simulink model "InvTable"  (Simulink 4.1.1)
settings: Solver=FixedStepDiscrete  StartTime=0.0  StopTime=inf  FixedStep=samplePeriod  RelTol=1e-3
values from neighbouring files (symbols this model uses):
  aHome = zeros(1, nAct)    [TableInit.m]    (also in displA2T.m = positT2A([0, 0, 0, 0, 0, 0], h); displT2A.m = positT2A([0, 0, 0, 0, 0, 0], h))
  bal = [[ 1 -1 -1  1  0  0  0  0]    [TableInit.m]
  flowCanon = 63090.2    [TableInit.m]    (also in initialize.m)
  gasConstant = 1.8    [TableInit.m]    (also in initialize.m)
  gee = 0    [TableInit.m]    (also in initialize.m = geeCanon / linAccelCanon * ~isempty(find(dof==3)))
  iactParamsX = [actParamsX, dfGain, solver]    [TableInit.m]
  iactParamsY = [actParamsY, dfGain, solver]    [TableInit.m]
  iactParamsZ = [actParamsZ, dfGain, solver]    [TableInit.m]
  inertia = [Ixx 0 0; 0 Iyy 0; 0 0 Izz]    [TableInit.m]    (also in initialize.m = inertia + inertiaP2Q([0 0 0], massA(i), cgA(:,i)-cg,  						)
  inertiaCanon = 0.1130    (= 0.113)    [TableInit.m]    (also in initialize.m = 0.00029264264)
  linAccelCanon = 9.8    [TableInit.m]    (also in accelA2T.m = h(11); accelT2A.m = h(11); Test.m = 9800; initialize.m = 9810)
  linVelocCanon = 10.0    (= 10)    [TableInit.m]    (also in Test.m; initialize.m = 1000)
  mass = 17300    [TableInit.m]    (also in initialize.m = ones(3, 1) * (sum(massA) + massT + massS))
  massCanon = 0.4535924e-06    (= 4.535924e-07)    [TableInit.m]    (also in initialize.m)
  maxOilVolume = volume * (1 - (precharge/supplyPress)^(1/gasConstant))    (= 316.850998915)    [TableInit.m]
  precharge = 1916    [TableInit.m]    (also in initialize.m = 2000)
  pumpFlow = 1.0e10    (= 10000000000)    [TableInit.m]    (also in initialize.m)
  rb_w = [-1525.00  3683.70 -3683.70  1525.00 -1000.00  1000.00 -1000.00  1000.00    [TableInit.m]    (also in positT2A.m = [-h1 -h5  h5  h1 -h1 -h1  h1  h1;           h5 -h1  h1 -h5  ; animation.m = self.R * rb_w)
  returnPress = 50    [TableInit.m]    (also in initialize.m)
  rgt = -rtg    [TableInit.m]
  roll = tbl(4)    [positT2A.m]    (also in animation.m = drot(1) * canon)
  rotAccelCanon = 1    [TableInit.m]    (also in accelA2T.m = h(14); accelT2A.m = h(14); Test.m; initialize.m = 0.0174532925199)
  rotForceCanon = 1000    [TableInit.m]    (also in forceA2T.m = h(15); Test.m; initialize.m)
  rotVelocCanon = 1    [TableInit.m]    (also in accelA2T.m = h(13); accelT2A.m = h(13); Test.m; initialize.m = 0.0174532925199)
  rt_t = [-1525.00  1214.70 -1214.70  1525.00 -1000.00  1000.00 -1000.00  1000.00    [TableInit.m]    (also in positT2A.m = [-h1    -h4-sh  h4+sh  h1    -h1    -h1     h1     h1;      )
  rtg = [0 0 cg]    [TableInit.m]    (also in initialize.m = cg)
  rtx_t = [rt_t topPlane.topLeft(:)  topPlane.topRight(:)                        topPlane.botRight(:) topPlane.botLeft(:)                         midPlane.topLeft(:)  midPlane.topRight(:)                        midPlane.botRight(:) midPlane.botLeft(:)                         botPlane.topLeft(:)  botPlane.topRight(:)                        botPlane.botRight(:) botPlane.botLeft(:)]    [TableInit.m]
  samplePeriod = 1/1024    (= 0.0009765625)    [TableInit.m]    (also in viewer.m = eval(getHeaderValue(header, 'DELTA_T')); initialize.m = 0.00048828125)
  volume = 1437    [TableInit.m]    (also in quake.m = volume / 231.0; initialize.m = 160)
  volumeCanon = 3785412.0    (= 3785412)    [TableInit.m]    (also in initialize.m)
undefined symbols (not defined in the file or in its folder): magnitude
libraries: aerospace x14, simulink3 x14, simulink_extras x1

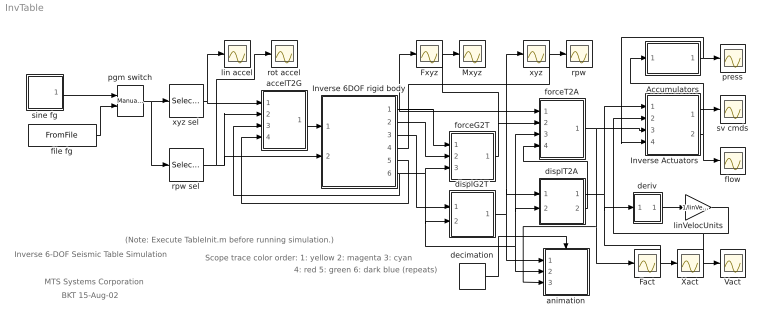
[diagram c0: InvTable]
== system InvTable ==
  note: Inverse 6-DOF Seismic Table Simulation
  note: BKT 15-Aug-02
  note: MTS Systems Corporation
  note: (Note: Execute TableInit.m before running simulation.)
  note: Scope trace color order: 1: yellow 2: magenta 3: cyan
  note: 4: red 5: green 6: dark blue (repeats)
  Accumulators : Subsystem
  Fact : Scope
  Fxyz : Scope
  Inverse 6DOF rigid body : Subsystem
  Inverse Actuators : Subsystem
  Mxyz : Scope
  Vact : Scope
  Xact : Scope
  accelT2G : Subsystem
  animation : Subsystem  TreatAsAtomicUnit=on  mask{type=2, azim=-37.5, elev=15}
      mask prompts: type "Drawing type (0: none, 1: wire frame, 2: solid)"; azim "View azimuth (degrees)"; elev "View elevation (degrees)"
  decimation : DiscretePulseGenerator  PulseType=Sample-based  Amplitude=1  Period=64  PulseWidth=1  PhaseDelay=0  SampleTime=samplePeriod
  deriv : Subsystem  mask{T=samplePeriod}
      mask prompts: T "Sample period (sec)"
  displG2T : Subsystem
  displT2A : Subsystem
  file fg : FromFile  FileName=KobeAccel.mat  SampleTime=samplePeriod
  flow : Scope
  forceG2T : Subsystem
  forceT2A : Subsystem
  lin accel : Scope
  linVelocUnits : Gain  Gain=1/linVelocCanon  Multiplication=Element-wise(K.*u)  SaturateOnIntegerOverflow=on
  pgm switch : simulink3/Nonlinear/Manual Switch  sw=1  action=0
  press : Scope
  rot accel : Scope
  rpw : Scope
  rpw sel : Selector  InputType=Vector  ElementSrc=Internal  Elements=[4 5 6]  RowSrc=Internal  Rows=1  ColumnSrc=Internal  Columns=1  InputPortWidth=6
  sine fg : Subsystem  mask(Sine Function Generator){dof=roll, ampl=200, freq=1, spanInterval=1}
      mask prompts: ampl "Amplitude"; freq "Frequency (Hz)"; spanInterval "Span interval (sec)"
  sv cmds : Scope
  xyz : Scope
  xyz sel : Selector  InputType=Vector  ElementSrc=Internal  Elements=[1 2 3]  RowSrc=Internal  Rows=1  ColumnSrc=Internal  Columns=1  InputPortWidth=6
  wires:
  xyz sel/1 -> lin accel/1, accelT2G/1(xyz)
  sine fg/1(out) -> pgm switch/1
  rpw sel/1 -> accelT2G/2(rpw), Inverse 6DOF rigid body/2(rot accel), rot accel/1
  accelT2G/1(out) -> Inverse 6DOF rigid body/1(lin accel)
  Inverse 6DOF rigid body/1(Fxyz) -> forceG2T/1(xyz), Fxyz/1, forceT2A/1(xyz)
  Inverse 6DOF rigid body/2(Mxyz) -> forceG2T/2(rpw)
  Inverse 6DOF rigid body/6(DCM) -> accelT2G/3(DCM), forceG2T/3(DCM), displG2T/2(DCM), displT2A/2(DCM), forceT2A/3(DCM), animation/2(DCM)
  forceG2T/1(out) -> Mxyz/1, forceT2A/2(rpw)
  displT2A/2(dir) -> forceT2A/4(dir)
  Inverse 6DOF rigid body/3(xyz) -> displG2T/1(xyz)
  Inverse 6DOF rigid body/5(rot veloc) -> accelT2G/4(rot veloc)
  displG2T/1(out) -> xyz/1, displT2A/1(xyz), animation/1(xyz)
  Inverse 6DOF rigid body/4(rpw) -> rpw/1
  deriv/1(out) -> linVelocUnits/1
  forceT2A/1(out) -> Inverse Actuators/3(force), Fact/1, animation/3(Fact)
  Inverse Actuators/1(cmd) -> sv cmds/1
  Inverse Actuators/2(flow) -> flow/1, Accumulators/1(flow)
  Accumulators/1(press) -> Inverse Actuators/4(press), press/1
  displT2A/1(out) -> Inverse Actuators/1(displ), Xact/1, deriv/1(inp)
  linVelocUnits/1 -> Inverse Actuators/2(veloc), Vact/1
  pgm switch/1 -> xyz sel/1, rpw sel/1
  file fg/1 -> pgm switch/2
  decimation/1 -> animation/Trigger

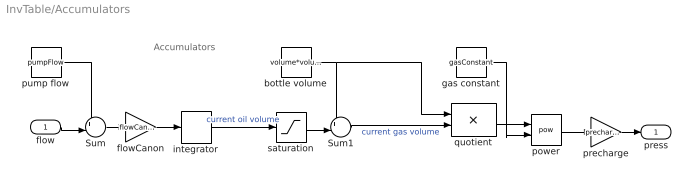
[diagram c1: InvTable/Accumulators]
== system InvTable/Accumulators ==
  note: Accumulators
  flow : Inport  Port=1  LatchInput=off
  Sum : Sum  Inputs=+-|  SaturateOnIntegerOverflow=on
  Sum1 : Sum  Inputs=+-|  SaturateOnIntegerOverflow=on
  bottle volume : Constant  Value=volume*volumeCanon
  flowCanon : Gain  Gain=flowCanon  Multiplication=Element-wise(K.*u)  SaturateOnIntegerOverflow=on
  gas constant : Constant  Value=gasConstant
  integrator : DiscreteIntegrator  IntegratorMethod=ForwardEuler  ExternalReset=none  InitialConditionSource=internal  InitialCondition=volume * (1 - (precharge/3000)^(1/gasConstant)) * 231  LimitOutput=off  UpperSaturationLimit=inf  LowerSaturationLimit=-inf  ShowSaturationPort=off  ShowStatePort=off  SampleTime=-1
  power : Math  Operator=pow  OutputSignalType=auto
  precharge : Gain  Gain=precharge  Multiplication=Element-wise(K.*u)  SaturateOnIntegerOverflow=on
  pump flow : Constant  Value=pumpFlow
  quotient : Product  Inputs=*/  Multiplication=Element-wise(.*)  SaturateOnIntegerOverflow=on
  saturation : Saturate  UpperLimit=maxOilVolume*volumeCanon  LowerLimit=0  LinearizeAsGain=on
  press : Outport  Port=1
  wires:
  pump flow/1 -> Sum/1
  Sum/1 -> flowCanon/1
  bottle volume/1 -> Sum1/1, quotient/1
  saturation/1 -> Sum1/2
  gas constant/1 -> power/2
  power/1 -> precharge/1
  precharge/1 -> press/1
  Sum1/1 -> quotient/2  "current gas volume"
  quotient/1 -> power/1
  integrator/1 -> saturation/1  "current oil volume"
  flow/1 -> Sum/2
  flowCanon/1 -> integrator/1

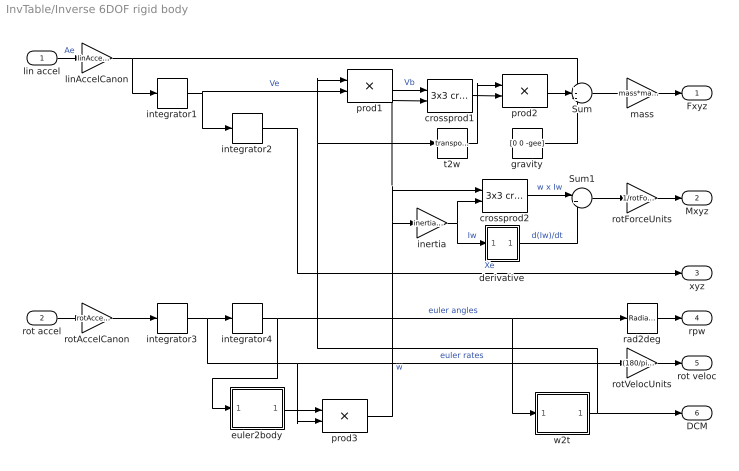
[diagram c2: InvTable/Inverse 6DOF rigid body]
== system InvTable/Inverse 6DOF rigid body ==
  lin accel : Inport  Port=1  LatchInput=off
  rot accel : Inport  Port=2  LatchInput=off
  Sum : Sum  Inputs=+--  SaturateOnIntegerOverflow=on
  Sum1 : Sum  Inputs=|++  SaturateOnIntegerOverflow=on
  crossprod1 : aerospace/Axes Transformations/3x3 cross product
  crossprod2 : aerospace/Axes Transformations/3x3 cross product
  derivative : Subsystem  mask{T=samplePeriod}
      mask prompts: T "Sample period (sec)"
  euler2body : Subsystem
  gravity : Constant  Value=[0 0 -gee]
  inertia : Gain  Gain=inertia*inertiaCanon  Multiplication=Matrix(K*u)  SaturateOnIntegerOverflow=on
  integrator{1..4} (4 alike) : DiscreteIntegrator  IntegratorMethod=ForwardEuler  ExternalReset=none  InitialConditionSource=internal  InitialCondition=0  LimitOutput=off  UpperSaturationLimit=inf  LowerSaturationLimit=-inf  ShowSaturationPort=off  ShowStatePort=off  SampleTime=-1
  linAccelCanon : Gain  Gain=linAccelCanon  Multiplication=Element-wise(K.*u)  SaturateOnIntegerOverflow=on
  mass : Gain  Gain=mass*massCanon  Multiplication=Element-wise(K.*u)  SaturateOnIntegerOverflow=on
  prod1 : Product  Inputs=2  Multiplication=Matrix(*)  SaturateOnIntegerOverflow=on
  prod2 : Product  Inputs=2  Multiplication=Matrix(*)  SaturateOnIntegerOverflow=on
  prod3 : Product  Inputs=2  Multiplication=Matrix(*)  SaturateOnIntegerOverflow=on
  rad2deg : simulink_extras/Transformations/Radians to Degrees
  rotAccelCanon : Gain  Gain=rotAccelCanon*(pi/180)  Multiplication=Element-wise(K.*u)  SaturateOnIntegerOverflow=on
  rotForceUnits : Gain  Gain=1/rotForceCanon  Multiplication=Element-wise(K.*u)  SaturateOnIntegerOverflow=on
  rotVelocUnits : Gain  Gain=(180/pi)/rotVelocCanon  Multiplication=Element-wise(K.*u)  SaturateOnIntegerOverflow=on
  t2w : Math  Operator=transpose  OutputSignalType=auto
  w2t : Subsystem
  Fxyz : Outport  Port=1
  Mxyz : Outport  Port=2
  xyz : Outport  Port=3
  rpw : Outport  Port=4
  rot veloc : Outport  Port=5
  DCM : Outport  Port=6
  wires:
  lin accel/1 -> linAccelCanon/1  "Ae"
  integrator1/1 -> prod1/2, integrator2/1  "Ve"
  Sum/1 -> mass/1
  gravity/1 -> Sum/3
  rot accel/1 -> rotAccelCanon/1
  inertia/1 -> crossprod2/2, derivative/1(inp)  "Iw"
  crossprod2/1 -> Sum1/1  "w x Iw"
  derivative/1(out) -> Sum1/2  "d(Iw)/dt"
  Sum1/1 -> rotForceUnits/1
  integrator2/1 -> xyz/1  "Xe"
  prod1/1 -> crossprod1/1  "Vb"
  mass/1 -> Fxyz/1
  crossprod1/1 -> prod2/2
  t2w/1 -> prod2/1
  prod2/1 -> Sum/2
  rotAccelCanon/1 -> integrator3/1
  rad2deg/1 -> rpw/1
  rotVelocUnits/1 -> rot veloc/1
  linAccelCanon/1 -> Sum/1, integrator1/1
  rotForceUnits/1 -> Mxyz/1
  euler2body/1(out) -> prod3/1
  w2t/1(DCM) -> DCM/1, t2w/1, prod1/1
  integrator3/1 -> integrator4/1, rotVelocUnits/1, prod3/2  "euler rates"
  prod3/1 -> inertia/1, crossprod1/2, crossprod2/1  "w"
  integrator4/1 -> euler2body/1(rpw), rad2deg/1, w2t/1(rpw)  "euler angles"

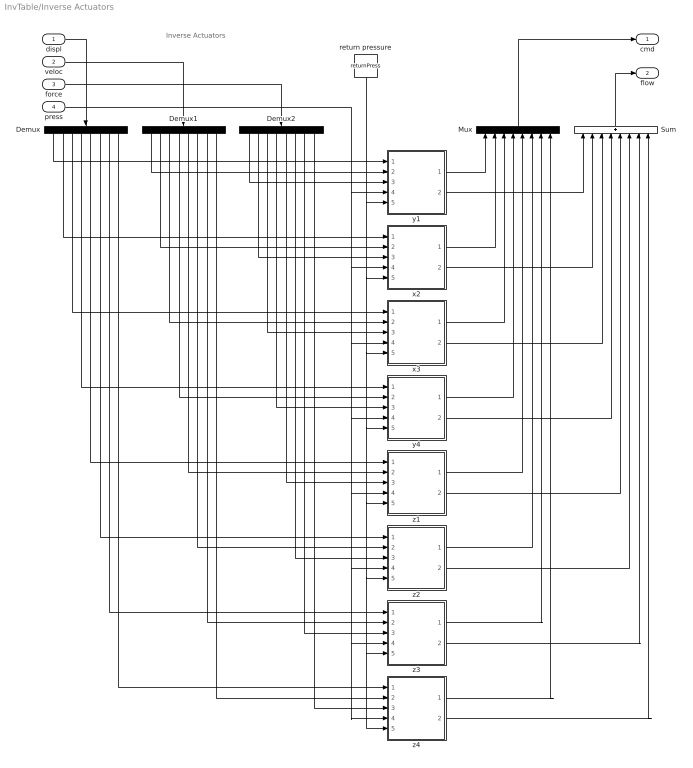
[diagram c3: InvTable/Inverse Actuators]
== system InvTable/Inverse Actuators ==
  note: Inverse Actuators
  displ : Inport  Port=1  LatchInput=off
  veloc : Inport  Port=2  LatchInput=off
  force : Inport  Port=3  LatchInput=off
  press : Inport  Port=4  LatchInput=off
  Demux : Demux  Orientation=down  Outputs=8  BusSelectionMode=off
  Demux1 : Demux  Orientation=down  Outputs=8  BusSelectionMode=off
  Demux2 : Demux  Orientation=down  Outputs=8  BusSelectionMode=off
  Mux : Mux  Orientation=up  Inputs=8
  Sum : Sum  Orientation=up  Inputs=8  SaturateOnIntegerOverflow=on
  return pressure : Constant  Orientation=down  Value=returnPress
  x2 : Subsystem  mask(Inverse Actuator){params=iactParamsX}
      mask prompts: params "Parameter vector"
  x3 : Subsystem  mask(Inverse Actuator){params=iactParamsX}
      mask prompts: params "Parameter vector"
  y1 : Subsystem  mask(Inverse Actuator){params=iactParamsY}
      mask prompts: params "Parameter vector"
  y4 : Subsystem  mask(Inverse Actuator){params=iactParamsY}
      mask prompts: params "Parameter vector"
  z1 : Subsystem  mask(Inverse Actuator){params=iactParamsZ}
      mask prompts: params "Parameter vector"
  z2 : Subsystem  mask(Inverse Actuator){params=iactParamsZ}
      mask prompts: params "Parameter vector"
  z3 : Subsystem  mask(Inverse Actuator){params=iactParamsZ}
      mask prompts: params "Parameter vector"
  z4 : Subsystem  mask(Inverse Actuator){params=iactParamsZ}
      mask prompts: params "Parameter vector"
  cmd : Outport  Port=1
  flow : Outport  Port=2
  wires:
  displ/1 -> Demux/1
  veloc/1 -> Demux1/1
  Demux/1 -> y1/1(displ)
  Demux/2 -> x2/1(displ)
  Demux1/1 -> y1/2(veloc)
  Demux2/1 -> y1/3(force)
  Demux1/2 -> x2/2(veloc)
  Demux2/2 -> x2/3(force)
  Demux/3 -> x3/1(displ)
  Demux1/3 -> x3/2(veloc)
  Demux2/3 -> x3/3(force)
  Demux/4 -> y4/1(displ)
  Demux1/4 -> y4/2(veloc)
  Demux2/4 -> y4/3(force)
  Demux/5 -> z1/1(displ)
  Demux1/5 -> z1/2(veloc)
  Demux2/5 -> z1/3(force)
  Demux/6 -> z2/1(displ)
  Demux1/6 -> z2/2(veloc)
  Demux2/6 -> z2/3(force)
  Demux/7 -> z3/1(displ)
  Demux1/7 -> z3/2(veloc)
  Demux2/7 -> z3/3(force)
  Demux/8 -> z4/1(displ)
  Demux1/8 -> z4/2(veloc)
  Demux2/8 -> z4/3(force)
  x3/1(cmd) -> Mux/3
  y4/1(cmd) -> Mux/4
  Mux/1 -> cmd/1
  z1/1(cmd) -> Mux/5
  z2/1(cmd) -> Mux/6
  z3/1(cmd) -> Mux/7
  z4/1(cmd) -> Mux/8
  force/1 -> Demux2/1
  y1/1(cmd) -> Mux/1
  x2/1(cmd) -> Mux/2
  y1/2(flow) -> Sum/1
  x2/2(flow) -> Sum/2
  x3/2(flow) -> Sum/3
  y4/2(flow) -> Sum/4
  z1/2(flow) -> Sum/5
  z2/2(flow) -> Sum/6
  z3/2(flow) -> Sum/7
  z4/2(flow) -> Sum/8
  Sum/1 -> flow/1
  press/1 -> z3/4(spl press), z4/4(spl press), z2/4(spl press), z1/4(spl press), y4/4(spl press), x3/4(spl press), x2/4(spl press), y1/4(spl press)
  return pressure/1 -> z3/5(rtn press), z4/5(rtn press), z2/5(rtn press), z1/5(rtn press), y4/5(rtn press), x3/5(rtn press), x2/5(rtn press), y1/5(rtn press)

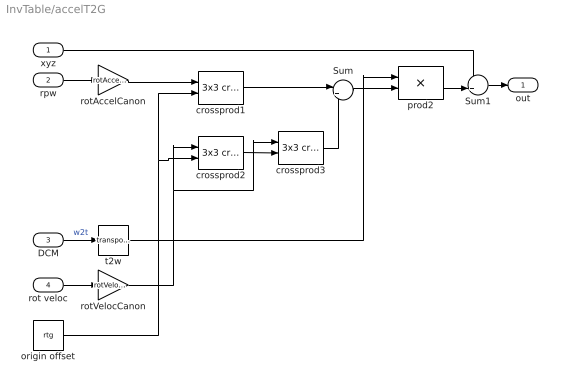
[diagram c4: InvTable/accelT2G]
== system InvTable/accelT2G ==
  xyz : Inport  Port=1  LatchInput=off
  rpw : Inport  Port=2  LatchInput=off
  DCM : Inport  Port=3  LatchInput=off
  rot veloc : Inport  Port=4  LatchInput=off
  Sum : Sum  Inputs=|++  SaturateOnIntegerOverflow=on
  Sum1 : Sum  Inputs=++|  SaturateOnIntegerOverflow=on
  crossprod1 : aerospace/Axes Transformations/3x3 cross product
  crossprod2 : aerospace/Axes Transformations/3x3 cross product
  crossprod3 : aerospace/Axes Transformations/3x3 cross product
  origin offset : Constant  Value=rtg
  prod2 : Product  Inputs=2  Multiplication=Matrix(*)  SaturateOnIntegerOverflow=on
  rotAccelCanon : Gain  Gain=rotAccelCanon*(pi/180)/linAccelCanon  Multiplication=Element-wise(K.*u)  SaturateOnIntegerOverflow=on
  rotVelocCanon : Gain  Gain=rotVelocCanon*(pi/180)/sqrt(linAccelCanon)  Multiplication=Element-wise(K.*u)  SaturateOnIntegerOverflow=on
  t2w : Math  Operator=transpose  OutputSignalType=auto
  out : Outport  Port=1
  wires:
  crossprod1/1 -> Sum/1
  crossprod3/1 -> Sum/2
  Sum1/1 -> out/1
  prod2/1 -> Sum1/2
  crossprod2/1 -> crossprod3/2
  Sum/1 -> prod2/2
  origin offset/1 -> crossprod1/2, crossprod2/2
  rotAccelCanon/1 -> crossprod1/1
  rpw/1 -> rotAccelCanon/1
  t2w/1 -> prod2/1
  xyz/1 -> Sum1/1
  rot veloc/1 -> rotVelocCanon/1
  DCM/1 -> t2w/1  "w2t"
  rotVelocCanon/1 -> crossprod3/1, crossprod2/1

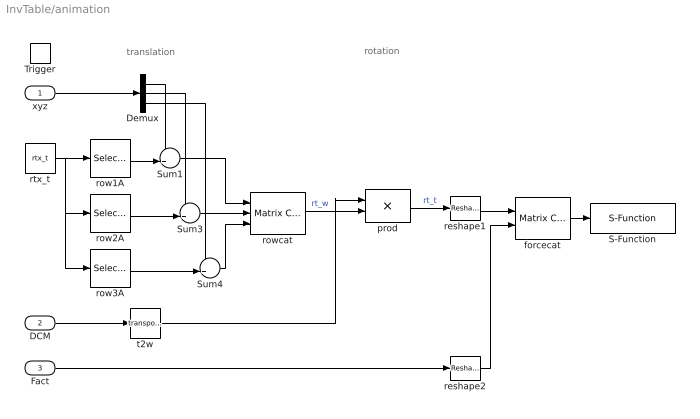
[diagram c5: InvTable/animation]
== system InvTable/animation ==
  note: translation
  note: rotation
  xyz : Inport  Port=1  LatchInput=off
  DCM : Inport  Port=2  LatchInput=off
  Fact : Inport  Port=3  LatchInput=off
  Trigger : TriggerPort  TriggerType=rising  OutputDataType=auto
  Demux : Demux  Outputs=3  BusSelectionMode=off
  S-Function : S-Function  FunctionName=tableAnimation  Parameters=type, rb_w, zmax,fmax,lines,faces,cmap,azim,elev  PortCounts=[]  SFunctionModules=''
  Sum1 : Sum  Inputs=-+|  SaturateOnIntegerOverflow=on
  Sum3 : Sum  Inputs=-+|  SaturateOnIntegerOverflow=on
  Sum4 : Sum  Inputs=-+|  SaturateOnIntegerOverflow=on
  forcecat : simulink3/Signals & Systems/Matrix Concatenation  numInports=2  catMethod=Vertical
  prod : Product  Inputs=2  Multiplication=Matrix(*)  SaturateOnIntegerOverflow=on
  reshape1 : simulink3/Signals & Systems/Reshape  OutputDimensionality=1-D array  OutputDimensions=[1,1]
  reshape2 : simulink3/Signals & Systems/Reshape  OutputDimensionality=1-D array  OutputDimensions=[1,1]
  row1A : Selector  InputType=Matrix  ElementSrc=Internal  Elements=[1 3]  RowSrc=Internal  Rows=1  ColumnSrc=Internal  Columns=-1  InputPortWidth=3
  row2A : Selector  InputType=Matrix  ElementSrc=Internal  Elements=[1 3]  RowSrc=Internal  Rows=2  ColumnSrc=Internal  Columns=-1  InputPortWidth=3
  row3A : Selector  InputType=Matrix  ElementSrc=Internal  Elements=[1 3]  RowSrc=Internal  Rows=3  ColumnSrc=Internal  Columns=-1  InputPortWidth=3
  rowcat : simulink3/Signals & Systems/Matrix Concatenation  numInports=3  catMethod=Vertical
  rtx_t : Constant  Value=rtx_t
  t2w : Math  Operator=transpose  OutputSignalType=auto
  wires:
  DCM/1 -> t2w/1
  xyz/1 -> Demux/1
  row1A/1 -> Sum1/2
  Demux/1 -> Sum1/1
  row2A/1 -> Sum3/2
  row3A/1 -> Sum4/2
  Demux/2 -> Sum3/1
  Demux/3 -> Sum4/1
  Sum3/1 -> rowcat/2
  Sum1/1 -> rowcat/1
  Sum4/1 -> rowcat/3
  t2w/1 -> prod/1
  rtx_t/1 -> row1A/1, row2A/1, row3A/1
  rowcat/1 -> prod/2  "rt_w"
  prod/1 -> reshape1/1  "rt_t"
  Fact/1 -> reshape2/1
  reshape1/1 -> forcecat/1
  forcecat/1 -> S-Function/1
  reshape2/1 -> forcecat/2

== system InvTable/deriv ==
  inp : Inport  Port=1  LatchInput=off
  1/T : Gain  Gain=1/T  Multiplication=Element-wise(K.*u)  SaturateOnIntegerOverflow=on
  Sum : Sum  Inputs=|+-  SaturateOnIntegerOverflow=on
  Unit Delay : UnitDelay  X0=0  SampleTime=-1
  out : Outport  Port=1
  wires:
  inp/1 -> Sum/1, Unit Delay/1
  Unit Delay/1 -> Sum/2
  Sum/1 -> 1/T/1
  1/T/1 -> out/1

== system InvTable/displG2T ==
  xyz : Inport  Port=1  LatchInput=off
  DCM : Inport  Port=2  LatchInput=off
  Sum1 : Sum  Inputs=+-+  SaturateOnIntegerOverflow=on
  origin offset : Constant  Value=rgt
  prod : Product  Inputs=2  Multiplication=Matrix(*)  SaturateOnIntegerOverflow=on
  out : Outport  Port=1
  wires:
  DCM/1 -> prod/1
  origin offset/1 -> prod/2, Sum1/3
  xyz/1 -> Sum1/1
  prod/1 -> Sum1/2
  Sum1/1 -> out/1

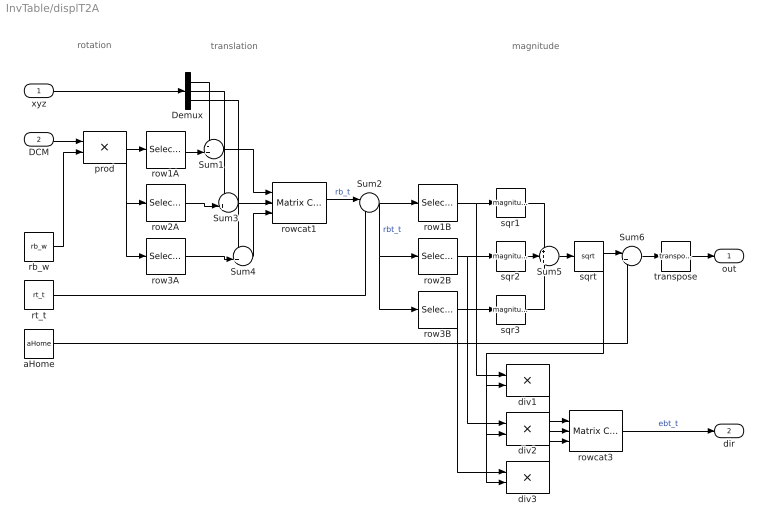
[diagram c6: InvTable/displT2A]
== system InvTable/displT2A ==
  note: rotation
  note: magnitude
  note: translation
  xyz : Inport  Port=1  LatchInput=off
  DCM : Inport  Port=2  LatchInput=off
  Demux : Demux  Outputs=3  BusSelectionMode=off
  Sum1 : Sum  Inputs=-+|  SaturateOnIntegerOverflow=on
  Sum2 : Sum  Inputs=|-+  SaturateOnIntegerOverflow=on
  Sum3 : Sum  Inputs=-+|  SaturateOnIntegerOverflow=on
  Sum4 : Sum  Inputs=-+|  SaturateOnIntegerOverflow=on
  Sum5 : Sum  Inputs=+++  SaturateOnIntegerOverflow=on
  Sum6 : Sum  Inputs=|+-  SaturateOnIntegerOverflow=on
  aHome : Constant  Value=aHome
  div1 : Product  Inputs=*/  Multiplication=Element-wise(.*)  SaturateOnIntegerOverflow=on
  div2 : Product  Inputs=*/  Multiplication=Element-wise(.*)  SaturateOnIntegerOverflow=on
  div3 : Product  Inputs=*/  Multiplication=Element-wise(.*)  SaturateOnIntegerOverflow=on
  prod : Product  Inputs=2  Multiplication=Matrix(*)  SaturateOnIntegerOverflow=on
  rb_w : Constant  Value=rb_w
  row1A : Selector  InputType=Matrix  ElementSrc=Internal  Elements=[1 3]  RowSrc=Internal  Rows=1  ColumnSrc=Internal  Columns=-1  InputPortWidth=3
  row1B : Selector  InputType=Matrix  ElementSrc=Internal  Elements=[1 3]  RowSrc=Internal  Rows=1  ColumnSrc=Internal  Columns=-1  InputPortWidth=3
  row2A : Selector  InputType=Matrix  ElementSrc=Internal  Elements=[1 3]  RowSrc=Internal  Rows=2  ColumnSrc=Internal  Columns=-1  InputPortWidth=3
  row2B : Selector  InputType=Matrix  ElementSrc=Internal  Elements=[1 3]  RowSrc=Internal  Rows=2  ColumnSrc=Internal  Columns=-1  InputPortWidth=3
  row3A : Selector  InputType=Matrix  ElementSrc=Internal  Elements=[1 3]  RowSrc=Internal  Rows=3  ColumnSrc=Internal  Columns=-1  InputPortWidth=3
  row3B : Selector  InputType=Matrix  ElementSrc=Internal  Elements=[1 3]  RowSrc=Internal  Rows=3  ColumnSrc=Internal  Columns=-1  InputPortWidth=3
  rowcat1 : simulink3/Signals & Systems/Matrix Concatenation  numInports=3  catMethod=Vertical
  rowcat3 : simulink3/Signals & Systems/Matrix Concatenation  numInports=3  catMethod=Vertical
  rt_t : Constant  Value=rt_t
  sqr1 : Math  Operator=magnitude^2  OutputSignalType=auto
  sqr2 : Math  Operator=magnitude^2  OutputSignalType=auto
  sqr3 : Math  Operator=magnitude^2  OutputSignalType=auto
  sqrt : Math  Operator=sqrt  OutputSignalType=auto
  transpose : Math  Operator=transpose  OutputSignalType=auto
  out : Outport  Port=1
  dir : Outport  Port=2
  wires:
  rb_w/1 -> prod/2
  prod/1 -> row1A/1, row3A/1, row2A/1
  xyz/1 -> Demux/1
  row1A/1 -> Sum1/2
  Demux/1 -> Sum1/1
  row2A/1 -> Sum3/2
  row3A/1 -> Sum4/2
  Demux/2 -> Sum3/1
  Demux/3 -> Sum4/1
  Sum3/1 -> rowcat1/2
  Sum1/1 -> rowcat1/1
  Sum4/1 -> rowcat1/3
  rt_t/1 -> Sum2/2
  row2B/1 -> sqr2/1, div2/1
  row1B/1 -> sqr1/1, div1/1
  row3B/1 -> sqr3/1, div3/1
  Sum5/1 -> sqrt/1
  aHome/1 -> Sum6/2
  sqrt/1 -> Sum6/1, div1/2, div2/2, div3/2
  rowcat1/1 -> Sum2/1  "rb_t"
  Sum2/1 -> row3B/1, row2B/1, row1B/1  "rbt_t"
  sqr1/1 -> Sum5/1
  sqr2/1 -> Sum5/2
  sqr3/1 -> Sum5/3
  rowcat3/1 -> dir/1  "ebt_t"
  div1/1 -> rowcat3/1
  div2/1 -> rowcat3/2
  div3/1 -> rowcat3/3
  DCM/1 -> prod/1
  Sum6/1 -> transpose/1
  transpose/1 -> out/1

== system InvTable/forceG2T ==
  xyz : Inport  Port=1  LatchInput=off
  rpw : Inport  Port=2  LatchInput=off
  DCM : Inport  Port=3  LatchInput=off
  Sum : Sum  Inputs=-+|  SaturateOnIntegerOverflow=on
  crossprod : aerospace/Axes Transformations/3x3 cross product
  origin offset : Constant  Value=rtg
  prod : Product  Inputs=2  Multiplication=Matrix(*)  SaturateOnIntegerOverflow=on
  rotForceUnits : Gain  Gain=1/rotForceCanon  Multiplication=Element-wise(K.*u)  SaturateOnIntegerOverflow=on
  out : Outport  Port=1
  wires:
  origin offset/1 -> crossprod/2
  prod/1 -> crossprod/1
  DCM/1 -> prod/1
  xyz/1 -> prod/2
  rotForceUnits/1 -> Sum/1
  crossprod/1 -> rotForceUnits/1
  Sum/1 -> out/1
  rpw/1 -> Sum/2

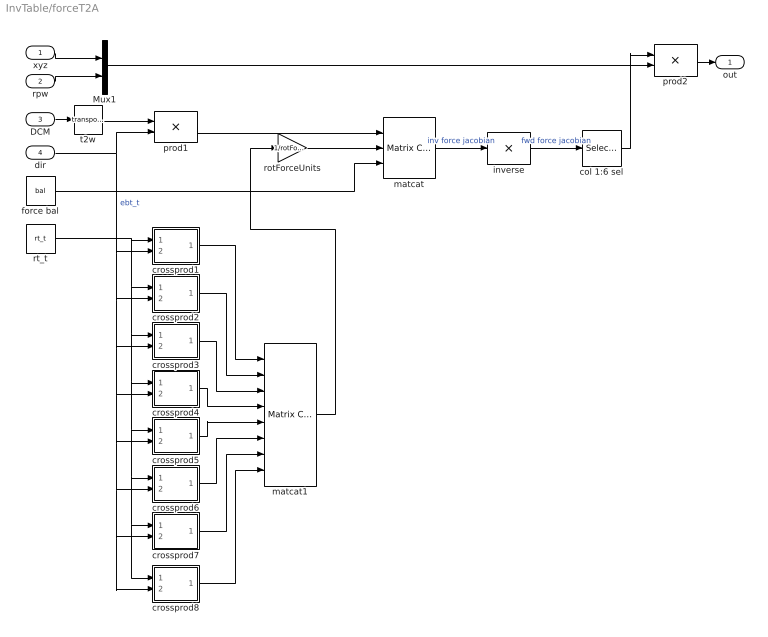
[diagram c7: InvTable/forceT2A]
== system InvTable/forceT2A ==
  xyz : Inport  Port=1  LatchInput=off
  rpw : Inport  Port=2  LatchInput=off
  DCM : Inport  Port=3  LatchInput=off
  dir : Inport  Port=4  LatchInput=off
  Mux1 : Mux  Inputs=2
  col 1:6 sel : Selector  InputType=Matrix  ElementSrc=Internal  Elements=[1 2 3 4 ]  RowSrc=Internal  Rows=-1  ColumnSrc=Internal  Columns=1:6  InputPortWidth=-1
  crossprod1 : Subsystem  mask{id=1}
      mask prompts: id "Actuator number"
  crossprod2 : Subsystem  mask{id=2}
      mask prompts: id "Actuator number"
  crossprod3 : Subsystem  mask{id=3}
      mask prompts: id "Actuator number"
  crossprod4 : Subsystem  mask{id=4}
      mask prompts: id "Actuator number"
  crossprod5 : Subsystem  mask{id=5}
      mask prompts: id "Actuator number"
  crossprod6 : Subsystem  mask{id=6}
      mask prompts: id "Actuator number"
  crossprod7 : Subsystem  mask{id=7}
      mask prompts: id "Actuator number"
  crossprod8 : Subsystem  mask{id=8}
      mask prompts: id "Actuator number"
  force bal : Constant  Value=bal
  inverse : Product  Inputs=/  Multiplication=Matrix(*)  SaturateOnIntegerOverflow=on
  matcat : simulink3/Signals & Systems/Matrix Concatenation  numInports=3  catMethod=Vertical
  matcat1 : simulink3/Signals & Systems/Matrix Concatenation  numInports=8  catMethod=Horizontal
  prod1 : Product  Inputs=2  Multiplication=Matrix(*)  SaturateOnIntegerOverflow=on
  prod2 : Product  Inputs=2  Multiplication=Matrix(*)  SaturateOnIntegerOverflow=on
  rotForceUnits : Gain  Gain=1/rotForceCanon  Multiplication=Element-wise(K.*u)  SaturateOnIntegerOverflow=on
  rt_t : Constant  Value=rt_t
  t2w : Math  Operator=transpose  OutputSignalType=auto
  out : Outport  Port=1
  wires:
  force bal/1 -> matcat/3
  t2w/1 -> prod1/1
  crossprod8/1(AxB) -> matcat1/8
  crossprod7/1(AxB) -> matcat1/7
  crossprod6/1(AxB) -> matcat1/6
  crossprod5/1(AxB) -> matcat1/5
  crossprod4/1(AxB) -> matcat1/4
  crossprod3/1(AxB) -> matcat1/3
  crossprod2/1(AxB) -> matcat1/2
  crossprod1/1(AxB) -> matcat1/1
  matcat1/1 -> rotForceUnits/1
  rt_t/1 -> crossprod2/1(A), crossprod3/1(A), crossprod4/1(A), crossprod5/1(A), crossprod6/1(A), crossprod8/1(A), crossprod7/1(A), crossprod1/1(A)
  prod1/1 -> matcat/1
  dir/1 -> crossprod2/2(B), crossprod3/2(B), crossprod4/2(B), crossprod5/2(B), crossprod6/2(B), crossprod8/2(B), crossprod7/2(B), crossprod1/2(B), prod1/2  "ebt_t"
  DCM/1 -> t2w/1
  matcat/1 -> inverse/1  "inv force jacobian"
  rotForceUnits/1 -> matcat/2
  prod2/1 -> out/1
  xyz/1 -> Mux1/1
  rpw/1 -> Mux1/2
  Mux1/1 -> prod2/2
  inverse/1 -> col 1:6 sel/1  "fwd force jacobian"
  col 1:6 sel/1 -> prod2/1

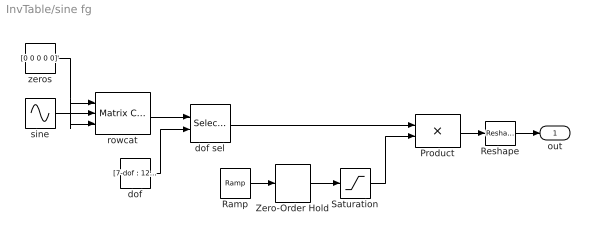
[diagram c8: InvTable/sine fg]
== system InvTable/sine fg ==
  Product : Product  Inputs=2  Multiplication=Element-wise(.*)  SaturateOnIntegerOverflow=on
  Ramp : simulink3/Sources/Ramp  slope=1/spanInterval  start=0  X0=0
  Reshape : simulink3/Signals & Systems/Reshape  OutputDimensionality=1-D array  OutputDimensions=[1,1]
  Saturation : Saturate  UpperLimit=1  LowerLimit=0  LinearizeAsGain=on
  Zero-Order Hold : ZeroOrderHold  SampleTime=samplePeriod
  dof : Constant  Value=[7-dof : 12-dof]
  dof sel : Selector  InputType=Vector  ElementSrc=External  Elements=-1  RowSrc=Internal  Rows=1  ColumnSrc=Internal  Columns=1  InputPortWidth=11
  rowcat : simulink3/Signals & Systems/Matrix Concatenation  numInports=3  catMethod=Vertical
  sine : Sin  SineType=Time-based  Amplitude=ampl  Bias=0  Frequency=2 * pi * freq  Phase=0  Samples=10  SampleTime=samplePeriod
  zeros : Constant  Value=[0 0 0 0 0]'
  out : Outport  Port=1
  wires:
  rowcat/1 -> dof sel/1
  zeros/1 -> rowcat/1, rowcat/3
  sine/1 -> rowcat/2
  dof/1 -> dof sel/2
  dof sel/1 -> Product/1
  Product/1 -> Reshape/1
  Ramp/1 -> Zero-Order Hold/1
  Zero-Order Hold/1 -> Saturation/1
  Saturation/1 -> Product/2
  Reshape/1 -> out/1

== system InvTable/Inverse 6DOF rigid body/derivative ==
  inp : Inport  Port=1  LatchInput=off
  1/T : Gain  Gain=1/T  Multiplication=Element-wise(K.*u)  SaturateOnIntegerOverflow=on
  Sum : Sum  Inputs=|+-  SaturateOnIntegerOverflow=on
  Unit Delay : UnitDelay  X0=0  SampleTime=-1
  out : Outport  Port=1
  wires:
  inp/1 -> Sum/1, Unit Delay/1
  Unit Delay/1 -> Sum/2
  Sum/1 -> 1/T/1
  1/T/1 -> out/1

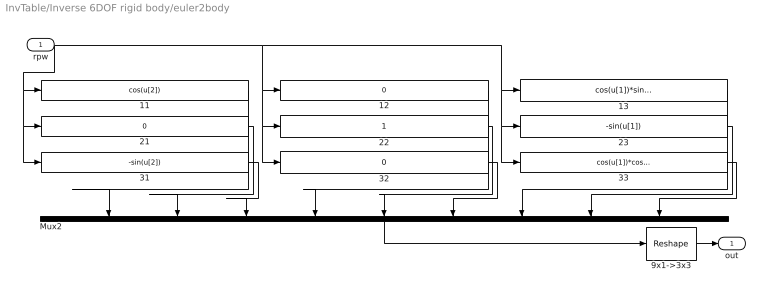
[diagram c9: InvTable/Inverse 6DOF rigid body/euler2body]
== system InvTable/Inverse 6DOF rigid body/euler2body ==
  rpw : Inport  Port=1  LatchInput=off
  11 : Fcn  Expr=cos(u[2])
  12 : Fcn  Expr=0
  13 : Fcn  Expr=cos(u[1])*sin(u[2])
  21 : Fcn  Expr=0
  22 : Fcn  Expr=1
  23 : Fcn  Expr=-sin(u[1])
  31 : Fcn  Expr=-sin(u[2])
  32 : Fcn  Expr=0
  33 : Fcn  Expr=cos(u[1])*cos(u[2])
  9x1->3x3 : simulink3/Signals & Systems/Reshape  OutputDimensionality=Customize  OutputDimensions=[3,3]
  Mux2 : Mux  Orientation=down  Inputs=9
  out : Outport  Port=1
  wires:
  33/1 -> Mux2/9
  23/1 -> Mux2/8
  13/1 -> Mux2/7
  Mux2/1 -> 9x1->3x3/1
  32/1 -> Mux2/6
  22/1 -> Mux2/5
  12/1 -> Mux2/4
  rpw/1 -> 13/1, 23/1, 33/1, 12/1, 22/1, 32/1, 11/1, 21/1, 31/1
  31/1 -> Mux2/3
  21/1 -> Mux2/2
  11/1 -> Mux2/1
  9x1->3x3/1 -> out/1

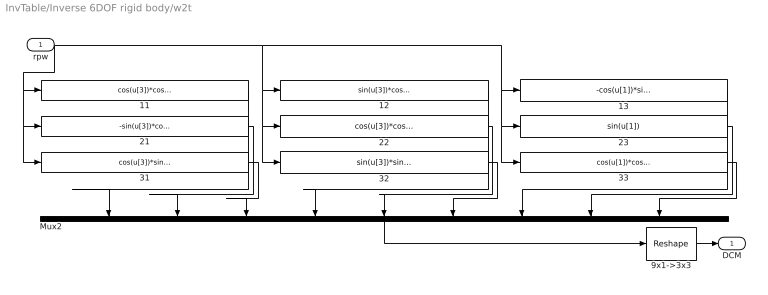
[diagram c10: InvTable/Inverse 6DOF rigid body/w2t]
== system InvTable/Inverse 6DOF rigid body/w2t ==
  rpw : Inport  Port=1  LatchInput=off
  11 : Fcn  Expr=cos(u[3])*cos(u[2])-sin(u[3])*sin(u[1])*sin(u[2])
  12 : Fcn  Expr=sin(u[3])*cos(u[2])+cos(u[3])*sin(u[1])*sin(u[2])
  13 : Fcn  Expr=-cos(u[1])*sin(u[2])
  21 : Fcn  Expr=-sin(u[3])*cos(u[1])
  22 : Fcn  Expr=cos(u[3])*cos(u[1])
  23 : Fcn  Expr=sin(u[1])
  31 : Fcn  Expr=cos(u[3])*sin(u[2])+sin(u[3])*sin(u[1])*cos(u[2])
  32 : Fcn  Expr=sin(u[3])*sin(u[2])-cos(u[3])*sin(u[1])*cos(u[2])
  33 : Fcn  Expr=cos(u[1])*cos(u[2])
  9x1->3x3 : simulink3/Signals & Systems/Reshape  OutputDimensionality=Customize  OutputDimensions=[3,3]
  Mux2 : Mux  Orientation=down  Inputs=9
  DCM : Outport  Port=1
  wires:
  9x1->3x3/1 -> DCM/1
  11/1 -> Mux2/1
  21/1 -> Mux2/2
  31/1 -> Mux2/3
  rpw/1 -> 31/1, 21/1, 11/1, 32/1, 22/1, 12/1, 33/1, 23/1, 13/1
  12/1 -> Mux2/4
  22/1 -> Mux2/5
  32/1 -> Mux2/6
  Mux2/1 -> 9x1->3x3/1
  13/1 -> Mux2/7
  23/1 -> Mux2/8
  33/1 -> Mux2/9

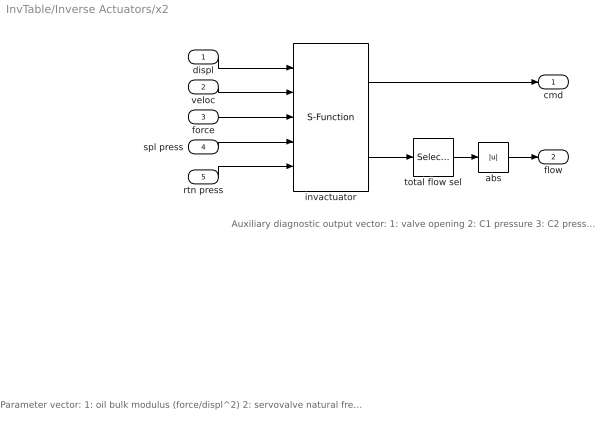
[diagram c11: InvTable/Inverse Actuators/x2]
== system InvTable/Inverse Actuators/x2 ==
  note: Auxiliary diagnostic output vector: 1: valve opening 2: C1 pressure 3: C2 pressure 4: delta pressure 5: force 6: velocity 7: C1 flow 8: C2 flow 9: total flow 10: kinematic flow 11: compressibility flow 12: leakage flow 13: iteration error
  note: Parameter vector: 1: oil bulk modulus (force/displ^2) 2: servovalve natural frequency (Hz) 3: servovalve damping ratio 4: servovalve overlap 5: rated pressure (force/displ^2) 6: flow at rated pressure (displ^3/sec) 7: actuator piston area 1 (displ^2) 8: actuator piston area 2 (displ^2) 9: actuator usable length (displ) 10: actuator endcap length (displ) 11: actuator parasitic damping factor 12: cross-chamber leakage factor (flow/press) 13: sample period (sec) Conversion factors used for converting signals from external (user) to internal (canonical) units: 14: displacement 15: velocity 16: force 17: pressure 18: flow Other: 19: delta-F feedback gain 20: inverse solver (0: exact, 1: approx)
  displ : Inport  Port=1  LatchInput=off
  veloc : Inport  Port=2  LatchInput=off
  force : Inport  Port=3  LatchInput=off
  spl press : Inport  Port=4  LatchInput=off
  rtn press : Inport  Port=5  LatchInput=off
  abs : Abs  SaturateOnIntegerOverflow=on
  invactuator : S-Function  FunctionName=invactuator  Parameters=params  PortCounts=[]  SFunctionModules=''
  total flow sel : Selector  InputType=Vector  ElementSrc=Internal  Elements=9  RowSrc=Internal  Rows=1  ColumnSrc=Internal  Columns=1  InputPortWidth=13
  cmd : Outport  Port=1
  flow : Outport  Port=2
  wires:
  abs/1 -> flow/1
  total flow sel/1 -> abs/1
  invactuator/2 -> total flow sel/1
  force/1 -> invactuator/3
  veloc/1 -> invactuator/2
  invactuator/1 -> cmd/1
  displ/1 -> invactuator/1
  rtn press/1 -> invactuator/5
  spl press/1 -> invactuator/4

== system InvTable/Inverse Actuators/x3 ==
  note: Parameter vector: 1: oil bulk modulus (force/displ^2) 2: servovalve natural frequency (Hz) 3: servovalve damping ratio 4: servovalve overlap 5: rated pressure (force/displ^2) 6: flow at rated pressure (displ^3/sec) 7: actuator piston area 1 (displ^2) 8: actuator piston area 2 (displ^2) 9: actuator usable length (displ) 10: actuator endcap length (displ) 11: actuator parasitic damping factor 12: cross-chamber leakage factor (flow/press) 13: sample period (sec) Conversion factors used for converting signals from external (user) to internal (canonical) units: 14: displacement 15: velocity 16: force 17: pressure 18: flow Other: 19: delta-F feedback gain 20: inverse solver (0: exact, 1: approx)
  note: Auxiliary diagnostic output vector: 1: valve opening 2: C1 pressure 3: C2 pressure 4: delta pressure 5: force 6: velocity 7: C1 flow 8: C2 flow 9: total flow 10: kinematic flow 11: compressibility flow 12: leakage flow 13: iteration error
  displ : Inport  Port=1  LatchInput=off
  veloc : Inport  Port=2  LatchInput=off
  force : Inport  Port=3  LatchInput=off
  spl press : Inport  Port=4  LatchInput=off
  rtn press : Inport  Port=5  LatchInput=off
  abs : Abs  SaturateOnIntegerOverflow=on
  invactuator : S-Function  FunctionName=invactuator  Parameters=params  PortCounts=[]  SFunctionModules=''
  total flow sel : Selector  InputType=Vector  ElementSrc=Internal  Elements=9  RowSrc=Internal  Rows=1  ColumnSrc=Internal  Columns=1  InputPortWidth=13
  cmd : Outport  Port=1
  flow : Outport  Port=2
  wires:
  spl press/1 -> invactuator/4
  rtn press/1 -> invactuator/5
  displ/1 -> invactuator/1
  invactuator/1 -> cmd/1
  veloc/1 -> invactuator/2
  force/1 -> invactuator/3
  invactuator/2 -> total flow sel/1
  total flow sel/1 -> abs/1
  abs/1 -> flow/1

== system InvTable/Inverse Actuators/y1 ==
  note: Parameter vector: 1: oil bulk modulus (force/displ^2) 2: servovalve natural frequency (Hz) 3: servovalve damping ratio 4: servovalve overlap 5: rated pressure (force/displ^2) 6: flow at rated pressure (displ^3/sec) 7: actuator piston area 1 (displ^2) 8: actuator piston area 2 (displ^2) 9: actuator usable length (displ) 10: actuator endcap length (displ) 11: actuator parasitic damping factor 12: cross-chamber leakage factor (flow/press) 13: sample period (sec) Conversion factors used for converting signals from external (user) to internal (canonical) units: 14: displacement 15: velocity 16: force 17: pressure 18: flow Other: 19: delta-F feedback gain 20: inverse solver (0: exact, 1: approx)
  note: Auxiliary diagnostic output vector: 1: valve opening 2: C1 pressure 3: C2 pressure 4: delta pressure 5: force 6: velocity 7: C1 flow 8: C2 flow 9: total flow 10: kinematic flow 11: compressibility flow 12: leakage flow 13: iteration error
  displ : Inport  Port=1  LatchInput=off
  veloc : Inport  Port=2  LatchInput=off
  force : Inport  Port=3  LatchInput=off
  spl press : Inport  Port=4  LatchInput=off
  rtn press : Inport  Port=5  LatchInput=off
  abs : Abs  SaturateOnIntegerOverflow=on
  invactuator : S-Function  FunctionName=invactuator  Parameters=params  PortCounts=[]  SFunctionModules=''
  total flow sel : Selector  InputType=Vector  ElementSrc=Internal  Elements=9  RowSrc=Internal  Rows=1  ColumnSrc=Internal  Columns=1  InputPortWidth=13
  cmd : Outport  Port=1
  flow : Outport  Port=2
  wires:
  spl press/1 -> invactuator/4
  rtn press/1 -> invactuator/5
  displ/1 -> invactuator/1
  invactuator/1 -> cmd/1
  veloc/1 -> invactuator/2
  force/1 -> invactuator/3
  invactuator/2 -> total flow sel/1
  total flow sel/1 -> abs/1
  abs/1 -> flow/1

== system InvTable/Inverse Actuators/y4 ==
  note: Auxiliary diagnostic output vector: 1: valve opening 2: C1 pressure 3: C2 pressure 4: delta pressure 5: force 6: velocity 7: C1 flow 8: C2 flow 9: total flow 10: kinematic flow 11: compressibility flow 12: leakage flow 13: iteration error
  note: Parameter vector: 1: oil bulk modulus (force/displ^2) 2: servovalve natural frequency (Hz) 3: servovalve damping ratio 4: servovalve overlap 5: rated pressure (force/displ^2) 6: flow at rated pressure (displ^3/sec) 7: actuator piston area 1 (displ^2) 8: actuator piston area 2 (displ^2) 9: actuator usable length (displ) 10: actuator endcap length (displ) 11: actuator parasitic damping factor 12: cross-chamber leakage factor (flow/press) 13: sample period (sec) Conversion factors used for converting signals from external (user) to internal (canonical) units: 14: displacement 15: velocity 16: force 17: pressure 18: flow Other: 19: delta-F feedback gain 20: inverse solver (0: exact, 1: approx)
  displ : Inport  Port=1  LatchInput=off
  veloc : Inport  Port=2  LatchInput=off
  force : Inport  Port=3  LatchInput=off
  spl press : Inport  Port=4  LatchInput=off
  rtn press : Inport  Port=5  LatchInput=off
  abs : Abs  SaturateOnIntegerOverflow=on
  invactuator : S-Function  FunctionName=invactuator  Parameters=params  PortCounts=[]  SFunctionModules=''
  total flow sel : Selector  InputType=Vector  ElementSrc=Internal  Elements=9  RowSrc=Internal  Rows=1  ColumnSrc=Internal  Columns=1  InputPortWidth=13
  cmd : Outport  Port=1
  flow : Outport  Port=2
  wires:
  abs/1 -> flow/1
  total flow sel/1 -> abs/1
  invactuator/2 -> total flow sel/1
  force/1 -> invactuator/3
  veloc/1 -> invactuator/2
  invactuator/1 -> cmd/1
  displ/1 -> invactuator/1
  rtn press/1 -> invactuator/5
  spl press/1 -> invactuator/4

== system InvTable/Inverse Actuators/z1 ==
  note: Parameter vector: 1: oil bulk modulus (force/displ^2) 2: servovalve natural frequency (Hz) 3: servovalve damping ratio 4: servovalve overlap 5: rated pressure (force/displ^2) 6: flow at rated pressure (displ^3/sec) 7: actuator piston area 1 (displ^2) 8: actuator piston area 2 (displ^2) 9: actuator usable length (displ) 10: actuator endcap length (displ) 11: actuator parasitic damping factor 12: cross-chamber leakage factor (flow/press) 13: sample period (sec) Conversion factors used for converting signals from external (user) to internal (canonical) units: 14: displacement 15: velocity 16: force 17: pressure 18: flow Other: 19: delta-F feedback gain 20: inverse solver (0: exact, 1: approx)
  note: Auxiliary diagnostic output vector: 1: valve opening 2: C1 pressure 3: C2 pressure 4: delta pressure 5: force 6: velocity 7: C1 flow 8: C2 flow 9: total flow 10: kinematic flow 11: compressibility flow 12: leakage flow 13: iteration error
  displ : Inport  Port=1  LatchInput=off
  veloc : Inport  Port=2  LatchInput=off
  force : Inport  Port=3  LatchInput=off
  spl press : Inport  Port=4  LatchInput=off
  rtn press : Inport  Port=5  LatchInput=off
  abs : Abs  SaturateOnIntegerOverflow=on
  invactuator : S-Function  FunctionName=invactuator  Parameters=params  PortCounts=[]  SFunctionModules=''
  total flow sel : Selector  InputType=Vector  ElementSrc=Internal  Elements=9  RowSrc=Internal  Rows=1  ColumnSrc=Internal  Columns=1  InputPortWidth=13
  cmd : Outport  Port=1
  flow : Outport  Port=2
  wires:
  spl press/1 -> invactuator/4
  rtn press/1 -> invactuator/5
  displ/1 -> invactuator/1
  invactuator/1 -> cmd/1
  veloc/1 -> invactuator/2
  force/1 -> invactuator/3
  invactuator/2 -> total flow sel/1
  total flow sel/1 -> abs/1
  abs/1 -> flow/1

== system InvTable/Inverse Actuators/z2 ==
  note: Auxiliary diagnostic output vector: 1: valve opening 2: C1 pressure 3: C2 pressure 4: delta pressure 5: force 6: velocity 7: C1 flow 8: C2 flow 9: total flow 10: kinematic flow 11: compressibility flow 12: leakage flow 13: iteration error
  note: Parameter vector: 1: oil bulk modulus (force/displ^2) 2: servovalve natural frequency (Hz) 3: servovalve damping ratio 4: servovalve overlap 5: rated pressure (force/displ^2) 6: flow at rated pressure (displ^3/sec) 7: actuator piston area 1 (displ^2) 8: actuator piston area 2 (displ^2) 9: actuator usable length (displ) 10: actuator endcap length (displ) 11: actuator parasitic damping factor 12: cross-chamber leakage factor (flow/press) 13: sample period (sec) Conversion factors used for converting signals from external (user) to internal (canonical) units: 14: displacement 15: velocity 16: force 17: pressure 18: flow Other: 19: delta-F feedback gain 20: inverse solver (0: exact, 1: approx)
  displ : Inport  Port=1  LatchInput=off
  veloc : Inport  Port=2  LatchInput=off
  force : Inport  Port=3  LatchInput=off
  spl press : Inport  Port=4  LatchInput=off
  rtn press : Inport  Port=5  LatchInput=off
  abs : Abs  SaturateOnIntegerOverflow=on
  invactuator : S-Function  FunctionName=invactuator  Parameters=params  PortCounts=[]  SFunctionModules=''
  total flow sel : Selector  InputType=Vector  ElementSrc=Internal  Elements=9  RowSrc=Internal  Rows=1  ColumnSrc=Internal  Columns=1  InputPortWidth=13
  cmd : Outport  Port=1
  flow : Outport  Port=2
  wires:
  abs/1 -> flow/1
  total flow sel/1 -> abs/1
  invactuator/2 -> total flow sel/1
  force/1 -> invactuator/3
  veloc/1 -> invactuator/2
  invactuator/1 -> cmd/1
  displ/1 -> invactuator/1
  rtn press/1 -> invactuator/5
  spl press/1 -> invactuator/4

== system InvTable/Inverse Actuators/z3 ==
  note: Parameter vector: 1: oil bulk modulus (force/displ^2) 2: servovalve natural frequency (Hz) 3: servovalve damping ratio 4: servovalve overlap 5: rated pressure (force/displ^2) 6: flow at rated pressure (displ^3/sec) 7: actuator piston area 1 (displ^2) 8: actuator piston area 2 (displ^2) 9: actuator usable length (displ) 10: actuator endcap length (displ) 11: actuator parasitic damping factor 12: cross-chamber leakage factor (flow/press) 13: sample period (sec) Conversion factors used for converting signals from external (user) to internal (canonical) units: 14: displacement 15: velocity 16: force 17: pressure 18: flow Other: 19: delta-F feedback gain 20: inverse solver (0: exact, 1: approx)
  note: Auxiliary diagnostic output vector: 1: valve opening 2: C1 pressure 3: C2 pressure 4: delta pressure 5: force 6: velocity 7: C1 flow 8: C2 flow 9: total flow 10: kinematic flow 11: compressibility flow 12: leakage flow 13: iteration error
  displ : Inport  Port=1  LatchInput=off
  veloc : Inport  Port=2  LatchInput=off
  force : Inport  Port=3  LatchInput=off
  spl press : Inport  Port=4  LatchInput=off
  rtn press : Inport  Port=5  LatchInput=off
  abs : Abs  SaturateOnIntegerOverflow=on
  invactuator : S-Function  FunctionName=invactuator  Parameters=params  PortCounts=[]  SFunctionModules=''
  total flow sel : Selector  InputType=Vector  ElementSrc=Internal  Elements=9  RowSrc=Internal  Rows=1  ColumnSrc=Internal  Columns=1  InputPortWidth=13
  cmd : Outport  Port=1
  flow : Outport  Port=2
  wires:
  spl press/1 -> invactuator/4
  rtn press/1 -> invactuator/5
  displ/1 -> invactuator/1
  invactuator/1 -> cmd/1
  veloc/1 -> invactuator/2
  force/1 -> invactuator/3
  invactuator/2 -> total flow sel/1
  total flow sel/1 -> abs/1
  abs/1 -> flow/1

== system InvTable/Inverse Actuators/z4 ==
  note: Auxiliary diagnostic output vector: 1: valve opening 2: C1 pressure 3: C2 pressure 4: delta pressure 5: force 6: velocity 7: C1 flow 8: C2 flow 9: total flow 10: kinematic flow 11: compressibility flow 12: leakage flow 13: iteration error
  note: Parameter vector: 1: oil bulk modulus (force/displ^2) 2: servovalve natural frequency (Hz) 3: servovalve damping ratio 4: servovalve overlap 5: rated pressure (force/displ^2) 6: flow at rated pressure (displ^3/sec) 7: actuator piston area 1 (displ^2) 8: actuator piston area 2 (displ^2) 9: actuator usable length (displ) 10: actuator endcap length (displ) 11: actuator parasitic damping factor 12: cross-chamber leakage factor (flow/press) 13: sample period (sec) Conversion factors used for converting signals from external (user) to internal (canonical) units: 14: displacement 15: velocity 16: force 17: pressure 18: flow Other: 19: delta-F feedback gain 20: inverse solver (0: exact, 1: approx)
  displ : Inport  Port=1  LatchInput=off
  veloc : Inport  Port=2  LatchInput=off
  force : Inport  Port=3  LatchInput=off
  spl press : Inport  Port=4  LatchInput=off
  rtn press : Inport  Port=5  LatchInput=off
  abs : Abs  SaturateOnIntegerOverflow=on
  invactuator : S-Function  FunctionName=invactuator  Parameters=params  PortCounts=[]  SFunctionModules=''
  total flow sel : Selector  InputType=Vector  ElementSrc=Internal  Elements=9  RowSrc=Internal  Rows=1  ColumnSrc=Internal  Columns=1  InputPortWidth=13
  cmd : Outport  Port=1
  flow : Outport  Port=2
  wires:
  abs/1 -> flow/1
  total flow sel/1 -> abs/1
  invactuator/2 -> total flow sel/1
  force/1 -> invactuator/3
  veloc/1 -> invactuator/2
  invactuator/1 -> cmd/1
  displ/1 -> invactuator/1
  rtn press/1 -> invactuator/5
  spl press/1 -> invactuator/4

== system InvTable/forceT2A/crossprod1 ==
  A : Inport  Port=1  LatchInput=off
  B : Inport  Port=2  LatchInput=off
  colA : Selector  InputType=Matrix  ElementSrc=Internal  Elements=[1 3]  RowSrc=Internal  Rows=-1  ColumnSrc=Internal  Columns=id  InputPortWidth=3
  colB : Selector  InputType=Matrix  ElementSrc=Internal  Elements=[1 3]  RowSrc=Internal  Rows=-1  ColumnSrc=Internal  Columns=id  InputPortWidth=3
  crossprod : aerospace/Axes Transformations/3x3 cross product
  AxB : Outport  Port=1
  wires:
  crossprod/1 -> AxB/1
  B/1 -> colB/1
  A/1 -> colA/1
  colB/1 -> crossprod/2
  colA/1 -> crossprod/1

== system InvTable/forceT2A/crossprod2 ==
  A : Inport  Port=1  LatchInput=off
  B : Inport  Port=2  LatchInput=off
  colA : Selector  InputType=Matrix  ElementSrc=Internal  Elements=[1 3]  RowSrc=Internal  Rows=-1  ColumnSrc=Internal  Columns=id  InputPortWidth=3
  colB : Selector  InputType=Matrix  ElementSrc=Internal  Elements=[1 3]  RowSrc=Internal  Rows=-1  ColumnSrc=Internal  Columns=id  InputPortWidth=3
  crossprod : aerospace/Axes Transformations/3x3 cross product
  AxB : Outport  Port=1
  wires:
  colA/1 -> crossprod/1
  colB/1 -> crossprod/2
  A/1 -> colA/1
  B/1 -> colB/1
  crossprod/1 -> AxB/1

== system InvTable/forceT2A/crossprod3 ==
  A : Inport  Port=1  LatchInput=off
  B : Inport  Port=2  LatchInput=off
  colA : Selector  InputType=Matrix  ElementSrc=Internal  Elements=[1 3]  RowSrc=Internal  Rows=-1  ColumnSrc=Internal  Columns=id  InputPortWidth=3
  colB : Selector  InputType=Matrix  ElementSrc=Internal  Elements=[1 3]  RowSrc=Internal  Rows=-1  ColumnSrc=Internal  Columns=id  InputPortWidth=3
  crossprod : aerospace/Axes Transformations/3x3 cross product
  AxB : Outport  Port=1
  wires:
  crossprod/1 -> AxB/1
  B/1 -> colB/1
  A/1 -> colA/1
  colB/1 -> crossprod/2
  colA/1 -> crossprod/1

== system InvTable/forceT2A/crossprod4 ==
  A : Inport  Port=1  LatchInput=off
  B : Inport  Port=2  LatchInput=off
  colA : Selector  InputType=Matrix  ElementSrc=Internal  Elements=[1 3]  RowSrc=Internal  Rows=-1  ColumnSrc=Internal  Columns=id  InputPortWidth=3
  colB : Selector  InputType=Matrix  ElementSrc=Internal  Elements=[1 3]  RowSrc=Internal  Rows=-1  ColumnSrc=Internal  Columns=id  InputPortWidth=3
  crossprod : aerospace/Axes Transformations/3x3 cross product
  AxB : Outport  Port=1
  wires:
  colA/1 -> crossprod/1
  colB/1 -> crossprod/2
  A/1 -> colA/1
  B/1 -> colB/1
  crossprod/1 -> AxB/1

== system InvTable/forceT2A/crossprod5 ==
  A : Inport  Port=1  LatchInput=off
  B : Inport  Port=2  LatchInput=off
  colA : Selector  InputType=Matrix  ElementSrc=Internal  Elements=[1 3]  RowSrc=Internal  Rows=-1  ColumnSrc=Internal  Columns=id  InputPortWidth=3
  colB : Selector  InputType=Matrix  ElementSrc=Internal  Elements=[1 3]  RowSrc=Internal  Rows=-1  ColumnSrc=Internal  Columns=id  InputPortWidth=3
  crossprod : aerospace/Axes Transformations/3x3 cross product
  AxB : Outport  Port=1
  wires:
  crossprod/1 -> AxB/1
  B/1 -> colB/1
  A/1 -> colA/1
  colB/1 -> crossprod/2
  colA/1 -> crossprod/1

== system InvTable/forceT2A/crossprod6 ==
  A : Inport  Port=1  LatchInput=off
  B : Inport  Port=2  LatchInput=off
  colA : Selector  InputType=Matrix  ElementSrc=Internal  Elements=[1 3]  RowSrc=Internal  Rows=-1  ColumnSrc=Internal  Columns=id  InputPortWidth=3
  colB : Selector  InputType=Matrix  ElementSrc=Internal  Elements=[1 3]  RowSrc=Internal  Rows=-1  ColumnSrc=Internal  Columns=id  InputPortWidth=3
  crossprod : aerospace/Axes Transformations/3x3 cross product
  AxB : Outport  Port=1
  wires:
  colA/1 -> crossprod/1
  colB/1 -> crossprod/2
  A/1 -> colA/1
  B/1 -> colB/1
  crossprod/1 -> AxB/1

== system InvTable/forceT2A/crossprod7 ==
  A : Inport  Port=1  LatchInput=off
  B : Inport  Port=2  LatchInput=off
  colA : Selector  InputType=Matrix  ElementSrc=Internal  Elements=[1 3]  RowSrc=Internal  Rows=-1  ColumnSrc=Internal  Columns=id  InputPortWidth=3
  colB : Selector  InputType=Matrix  ElementSrc=Internal  Elements=[1 3]  RowSrc=Internal  Rows=-1  ColumnSrc=Internal  Columns=id  InputPortWidth=3
  crossprod : aerospace/Axes Transformations/3x3 cross product
  AxB : Outport  Port=1
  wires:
  crossprod/1 -> AxB/1
  B/1 -> colB/1
  A/1 -> colA/1
  colB/1 -> crossprod/2
  colA/1 -> crossprod/1

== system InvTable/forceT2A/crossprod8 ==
  A : Inport  Port=1  LatchInput=off
  B : Inport  Port=2  LatchInput=off
  colA : Selector  InputType=Matrix  ElementSrc=Internal  Elements=[1 3]  RowSrc=Internal  Rows=-1  ColumnSrc=Internal  Columns=id  InputPortWidth=3
  colB : Selector  InputType=Matrix  ElementSrc=Internal  Elements=[1 3]  RowSrc=Internal  Rows=-1  ColumnSrc=Internal  Columns=id  InputPortWidth=3
  crossprod : aerospace/Axes Transformations/3x3 cross product
  AxB : Outport  Port=1
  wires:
  colA/1 -> crossprod/1
  colB/1 -> crossprod/2
  A/1 -> colA/1
  B/1 -> colB/1
  crossprod/1 -> AxB/1
